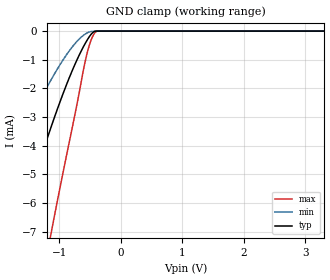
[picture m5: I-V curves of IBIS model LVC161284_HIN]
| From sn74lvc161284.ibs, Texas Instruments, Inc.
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[Model]   LVC161284_HIN
Model_type  Input
Vinl=1.6
Vinh=2.6
| variable   typ   min   max
C_comp   0.70pF   0.49pF   0.93pF
[Temperature Range]   40   100   -40
| Ambient temperature   25   85   -40
[Voltage range]   3.3   3   3.6
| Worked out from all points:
|   GND clamp passes 1 mA (typ) near -0.71 V on its own axis
[GND Clamp]
| LVC161284_HIN
|   Voltage   I(typ)   I(min)   I(max)
-5.5V     -38.52mA   -24.66mA   -66.57mA
-2.3V     -11.74mA   -7.062mA   -21.51mA
-2.22V    -11.12mA   -6.656mA   -20.45mA
-1.72V    -7.338mA   -4.213mA   -14.01mA
-1.655V   -6.866mA   -3.91mA    -13.2mA
-1.38V    -4.936mA   -2.685mA   -9.858mA
-1.13V    -3.303mA   -1.673mA   -6.976mA
-845mV    -1.65mA    -702.3uA   -3.914mA
-580mV    -426uA     -102.5uA   -1.042mA
-490mV    -124.6uA   -17.86uA   -339.5uA
-405mV    -112.8nA   -5.339uA   -20.87uA
3.3V      12.33pA    77.49pA    9.9pA
